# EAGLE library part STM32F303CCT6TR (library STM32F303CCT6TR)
ARM Microcontrollers - MCU Mainstream Mixed signals MCUs ARM Cortex-M4 core with DSP and FPU, 256 Kbytes Flash, 72 MHz CPU, MPU, CCM, 12-bit ADC 5 MSPS, PGA, comparators Source: Datasheet
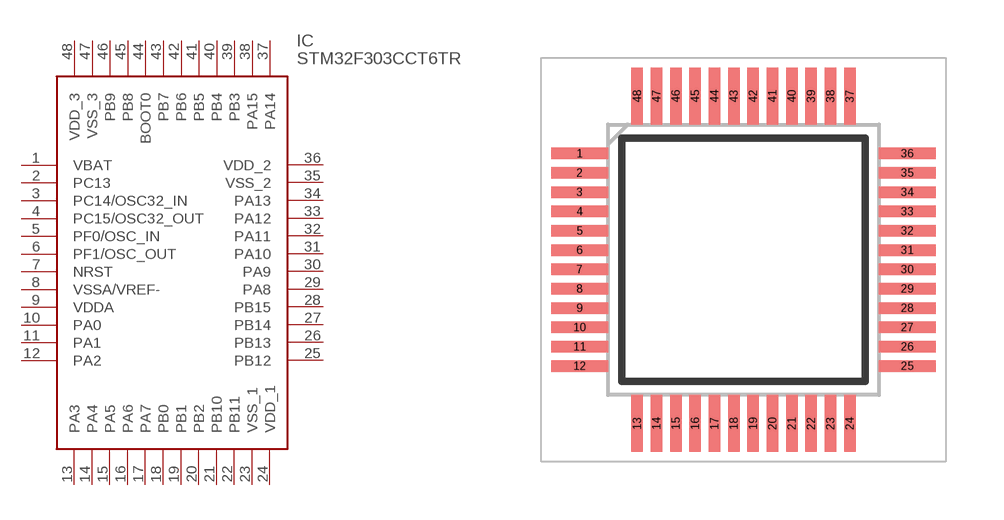
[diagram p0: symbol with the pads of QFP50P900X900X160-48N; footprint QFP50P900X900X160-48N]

Designator prefix IC

## STM32F303CCT6TR (Description: ARM Microcontrollers - MCU Mainstream Mixed signals MCUs ARM Cortex-M4 core with DSP and FPU, 256 Kbytes Flash, 72 MHz CPU, MPU, CCM, 12-bit ADC 5 MSPS, PGA, comparators; Height: 1.6mm; Manufacturer_Name: STMicroelectronics; Manufacturer_Part_Number: STM32F303CCT6TR; Mouser_Part_Number: 511-STM32F303CCT6TR; Mouser_Price-Stock: https://www.mouser.co.uk/ProductDetail/STMicroelectronics/STM32F303CCT6TR?qs=4b8myOmUP%252Bv8DFDnXNg9BQ%3D%3D)  [QFP50P900X900X160-48N]
1  VBAT
2  PC13
3  PC14/OSC32_IN
4  PC15/OSC32_OUT
5  PF0/OSC_IN
6  PF1/OSC_OUT
7  NRST
8  VSSA/VREF-
9  VDDA
10  PA0
11  PA1
12  PA2
13  PA3
14  PA4
15  PA5
16  PA6
17  PA7
18  PB0
19  PB1
20  PB2
21  PB10
22  PB11
23  VSS_1
24  VDD_1
25  PB12
26  PB13
27  PB14
28  PB15
29  PA8
30  PA9
31  PA10
32  PA11
33  PA12
34  PA13
35  VSS_2
36  VDD_2
37  PA14
38  PA15
39  PB3
40  PB4
41  PB5
42  PB6
43  PB7
44  BOOT0
45  PB8
46  PB9
47  VSS_3
48  VDD_3

## Footprint QFP50P900X900X160-48N (pad centres in mm)
LQFP48 - 48-pin, 7 x 7 mm
smd 1.475 x 0.3: 1 -4.238,2.75; 2 -4.238,2.25; 3 -4.238,1.75; 4 -4.238,1.25; 5 -4.238,0.75; 6 -4.238,0.25; 7 -4.238,-0.25; 8 -4.238,-0.75; 9 -4.238,-1.25; 10 -4.238,-1.75; 11 -4.238,-2.25; 12 -4.238,-2.75; 25 4.238,-2.75; 26 4.238,-2.25; 27 4.238,-1.75; 28 4.238,-1.25; 29 4.238,-0.75; 30 4.238,-0.25; 31 4.238,0.25; 32 4.238,0.75; 33 4.238,1.25; 34 4.238,1.75; 35 4.238,2.25; 36 4.238,2.75
smd 0.3 x 1.475: 13 -2.75,-4.238; 14 -2.25,-4.238; 15 -1.75,-4.238; 16 -1.25,-4.238; 17 -0.75,-4.238; 18 -0.25,-4.238; 19 0.25,-4.238; 20 0.75,-4.238; 21 1.25,-4.238; 22 1.75,-4.238; 23 2.25,-4.238; 24 2.75,-4.238; 37 2.75,4.238; 38 2.25,4.238; 39 1.75,4.238; 40 1.25,4.238; 41 0.75,4.238; 42 0.25,4.238; 43 -0.25,4.238; 44 -0.75,4.238; 45 -1.25,4.238; 46 -1.75,4.238; 47 -2.25,4.238; 48 -2.75,4.238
